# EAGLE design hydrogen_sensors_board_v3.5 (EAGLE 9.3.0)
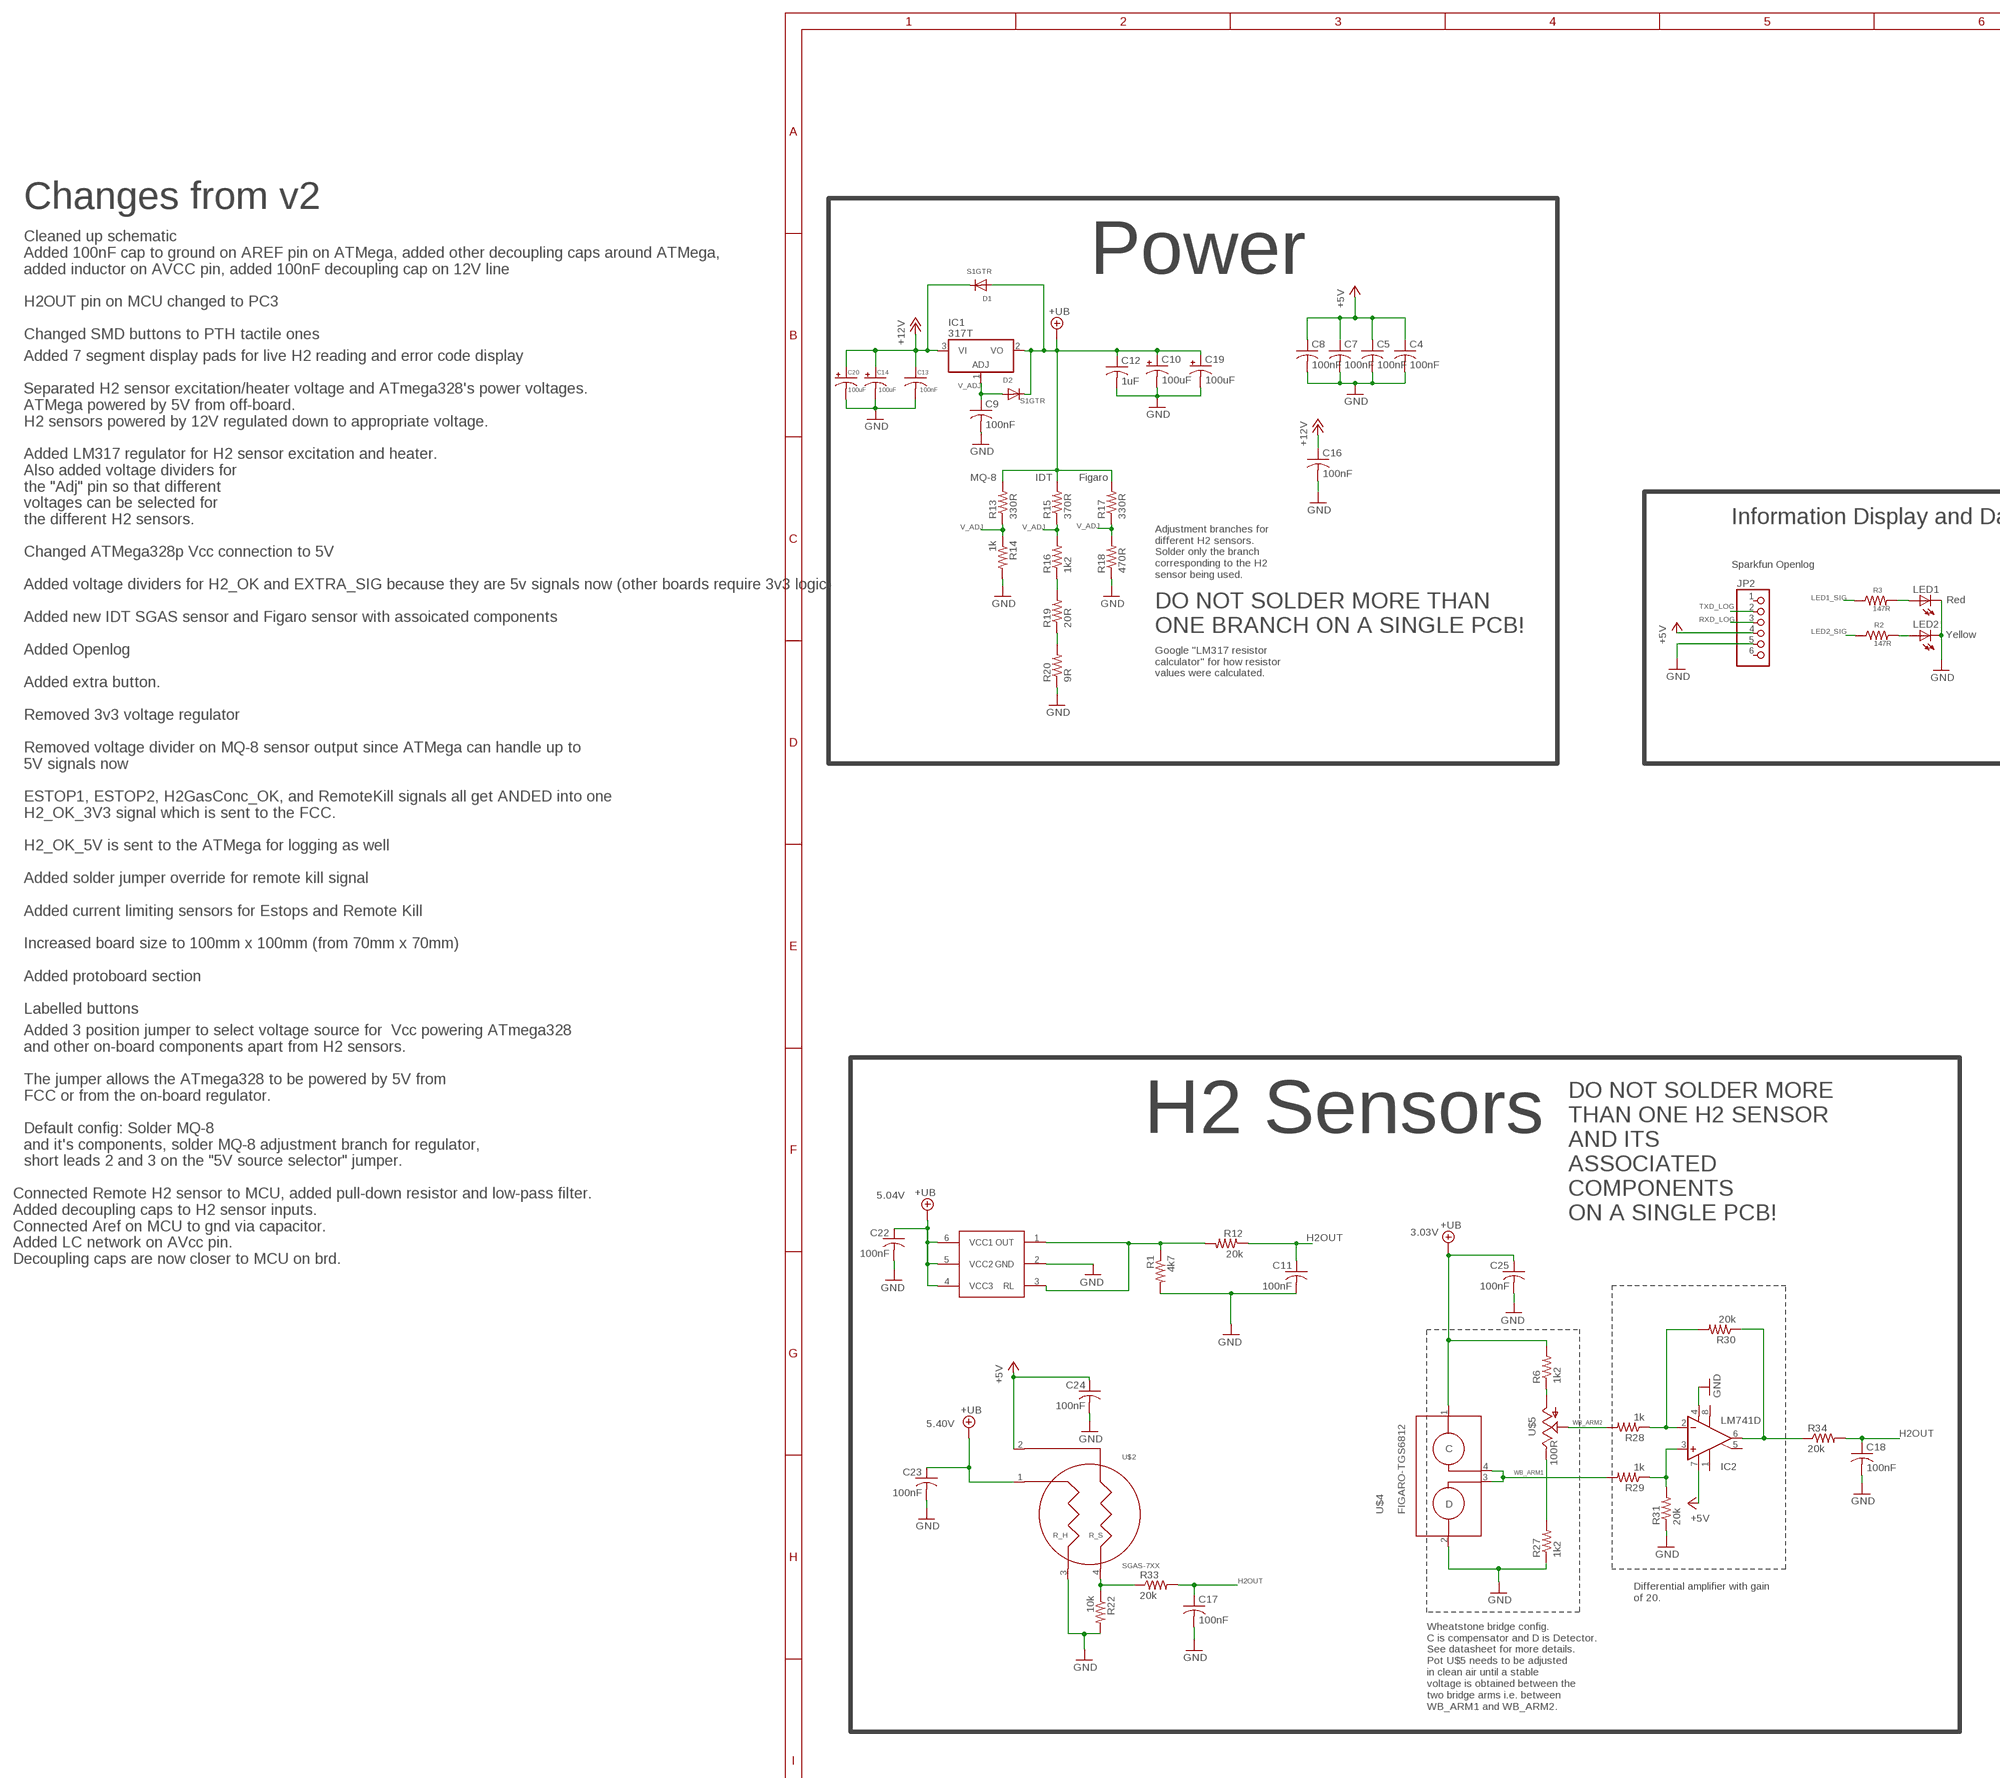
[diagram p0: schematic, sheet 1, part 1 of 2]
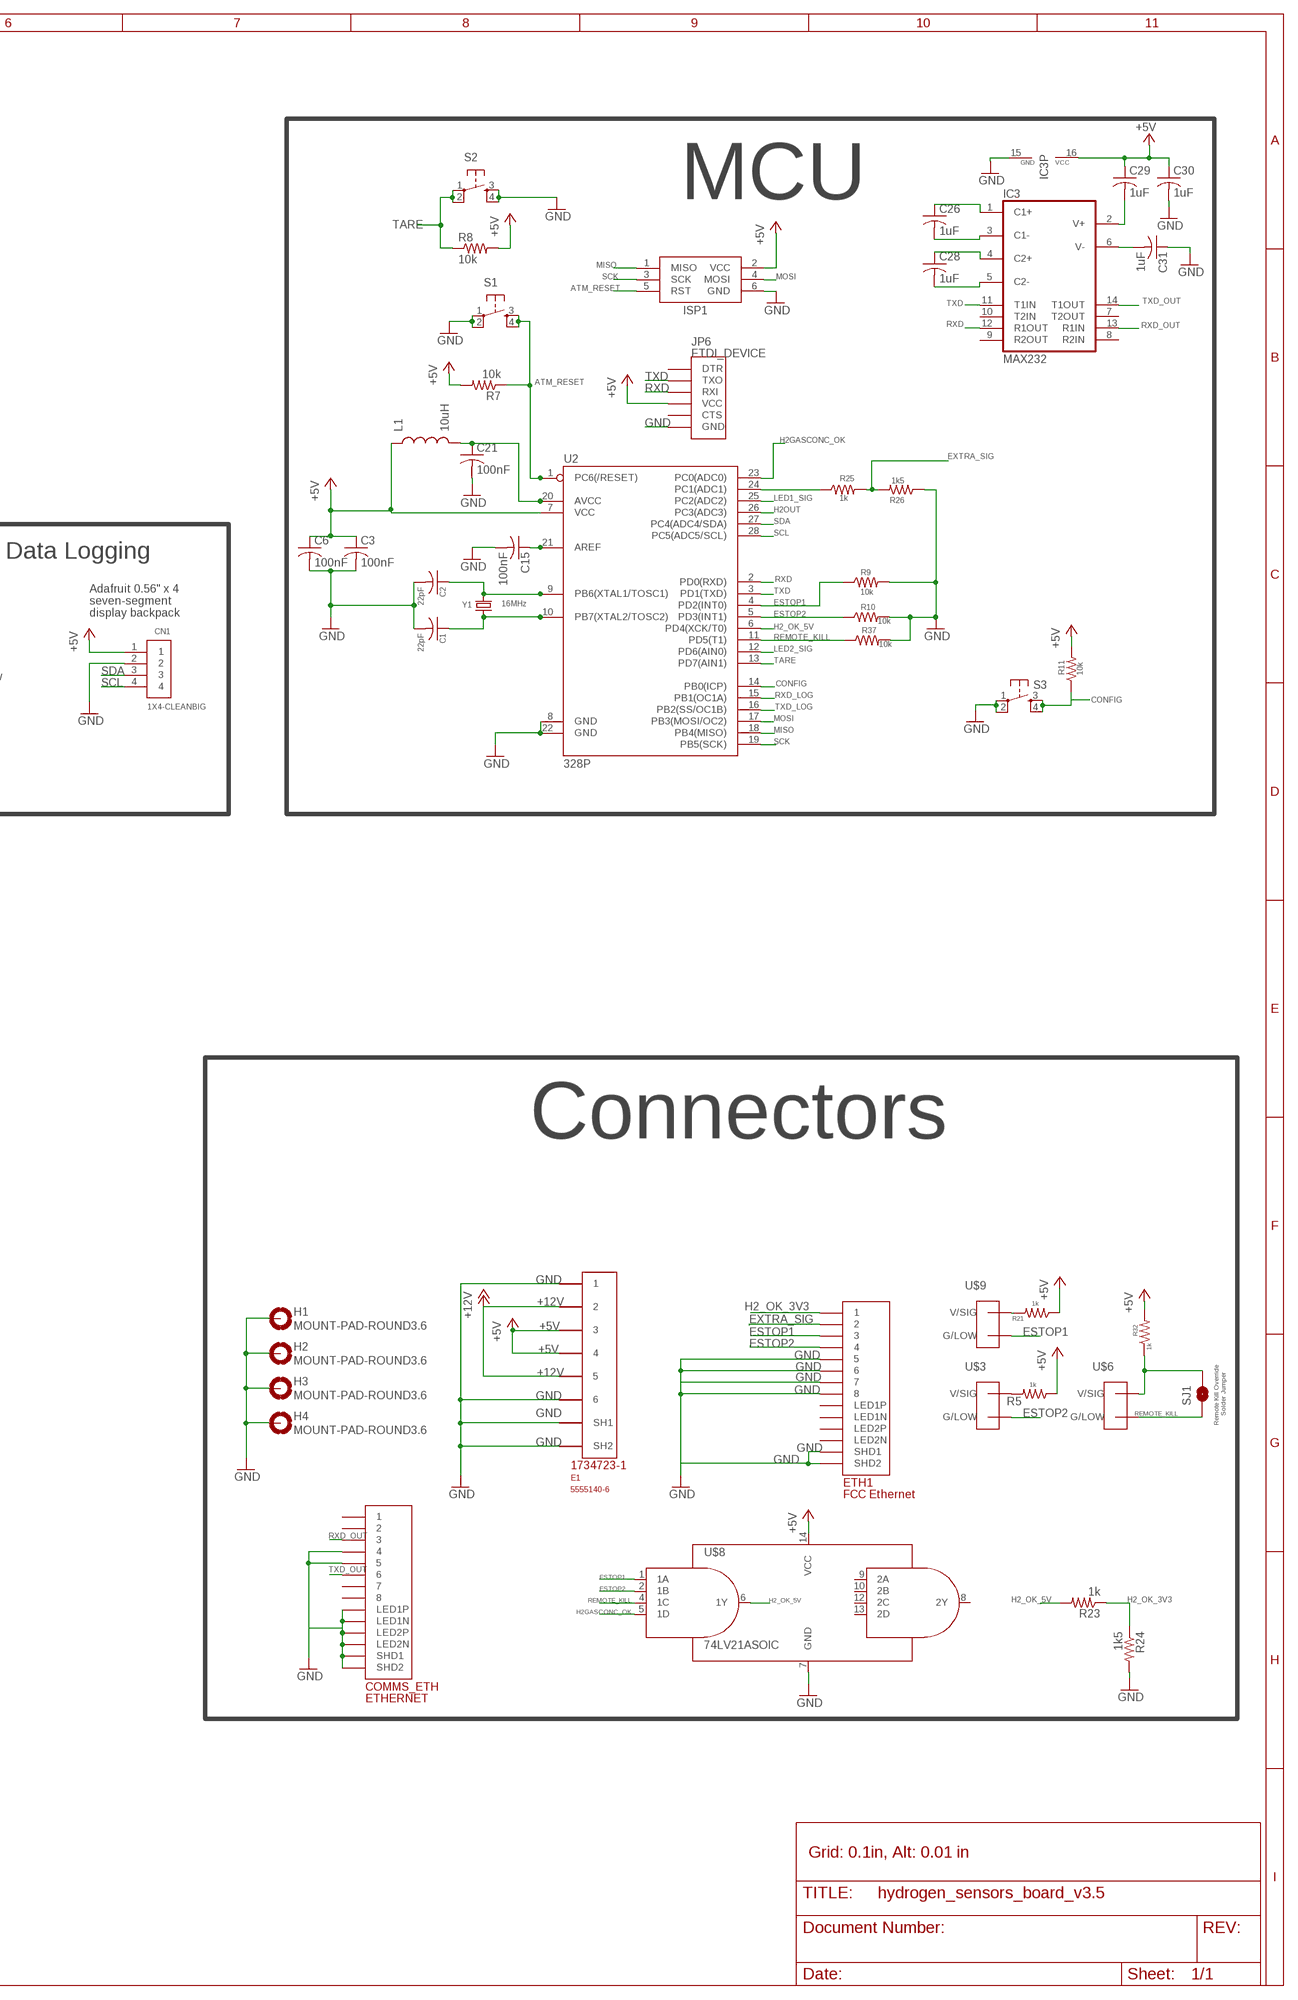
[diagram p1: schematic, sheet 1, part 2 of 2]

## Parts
C1  22pF  C-USC0603K  [C0603K]
C2  22pF  C-USC0603K  [C0603K]
C3  100nF  C-USC0603  [C0603]
C4  100nF  C-USC0603  [C0603]
C5  100nF  C-USC0603  [C0603]
C6  100nF  C-USC0603  [C0603]
C7  100nF  C-USC0603  [C0603]
C8  100nF  C-USC0603  [C0603]
C9  100nF  C-USC0603  [C0603]
C10  100uF  CPOL-USB/3528-21R  [B/3528-21R]
C11  100nF  C-USC0603  [C0603]
C12  1uF  C-USC0603  [C0603]
C13  100nF  C-USC0603  [C0603]
C14  100uF  CPOL-USB/3528-21R  [B/3528-21R]
C15  100nF  C-USC0603  [C0603]
C16  100nF  C-USC0603  [C0603]
C17  100nF  C-USC0603  [C0603]
C18  100nF  C-USC0603  [C0603]
C19  100uF  CAP_POLPTH1  [CPOL-RADIAL-100UF-25V]
C20  100uF  CAP_POLPTH1  [CPOL-RADIAL-100UF-25V]
C21  100nF  C-USC0603  [C0603]
C22  100nF  C-USC0603  [C0603]
C23  100nF  C-USC0603  [C0603]
C24  100nF  C-USC0603  [C0603]
C25  100nF  C-USC0603  [C0603]
C26  1uF  C-USC0603  [C0603]
C28  1uF  C-USC0603  [C0603]
C29  1uF  C-USC0603  [C0603]
C30  1uF  C-USC0603  [C0603]
C31  1uF  C-USC0603  [C0603]
CN1  1X4-CLEANBIG  [1X04-CLEANBIG]
COMMS_ETH  ETHERNET  [A122645-ND]
D1  S1GTR  DIODESMA  [SMADIODE]
D2  S1GTR  DIODESMA  [SMADIODE]
E1  5555140-6  [1734723-1_RJ11]
ETH1  FCC Ethernet  ETHERNET  [A122645-ND]
H1  MOUNT-PAD-ROUND3.6  [3,6-PAD]
H2  MOUNT-PAD-ROUND3.6  [3,6-PAD]
H3  MOUNT-PAD-ROUND3.6  [3,6-PAD]
H4  MOUNT-PAD-ROUND3.6  [3,6-PAD]
IC1  317T  [TO220H]
IC2  LM741D  [SO08]
IC3  MAX232  [DIL16]
ISP1  AVRISP-BOX  [AVRISP-BOX]
JP2  PINHD-1X6LOCK  [1X06-BIGLOCK]
JP6  FTDI_DEVICE  [FTDI_DEVICE_SIDE]
L1  10uH  INDUCTOR0603  [0603]
LED1  Red  LEDCHIPLED_0805  [CHIPLED_0805]
LED2  Yellow  LEDCHIPLED_0805  [CHIPLED_0805]
R1  4k7  RESISTOR0603-RES  [0603-RES]
R2  147R  RESISTOR0603-RES  [0603-RES]
R3  147R  RESISTOR0603-RES  [0603-RES]
R5  1k  RESISTOR0603-RES  [0603-RES]
R6  1k2  RESISTOR0603-RES  [0603-RES]
R7  10k  RESISTOR0603-RES  [0603-RES]
R8  10k  RESISTOR0603-RES  [0603-RES]
R9  10k  RESISTOR0603-RES  [0603-RES]
R10  10k  RESISTOR0603-RES  [0603-RES]
R11  10k  RESISTOR0603-RES  [0603-RES]
R12  20k  RESISTOR0603-RES  [0603-RES]
R13  330R  RESISTOR0603-RES  [0603-RES]
R14  1k  RESISTOR0603-RES  [0603-RES]
R15  370R  RESISTOR0603-RES  [0603-RES]
R16  1k2  RESISTOR0603-RES  [0603-RES]
R17  330R  RESISTOR0603-RES  [0603-RES]
R18  470R  RESISTOR0603-RES  [0603-RES]
R19  20R  RESISTOR0603-RES  [0603-RES]
R20  9R  RESISTOR0603-RES  [0603-RES]
R21  1k  RESISTOR0603-RES  [0603-RES]
R22  10k  RESISTOR0603-RES  [0603-RES]
R23  1k  RESISTOR0603-RES  [0603-RES]
R24  1k5  RESISTOR0603-RES  [0603-RES]
R25  1k  RESISTOR0603-RES  [0603-RES]
R26  1k5  RESISTOR0603-RES  [0603-RES]
R27  1k2  RESISTOR0603-RES  [0603-RES]
R28  1k  RESISTOR0603-RES  [0603-RES]
R29  1k  RESISTOR0603-RES  [0603-RES]
R30  20k  RESISTOR0603-RES  [0603-RES]
R31  20k  RESISTOR0603-RES  [0603-RES]
R32  1k  RESISTOR0603-RES  [0603-RES]
R33  20k  RESISTOR0603-RES  [0603-RES]
R34  20k  RESISTOR0603-RES  [0603-RES]
R37  10k  RESISTOR0603-RES  [0603-RES]
S1  TAC_SWITCHPTH  [TACTILE-PTH]
S2  TAC_SWITCHPTH  [TACTILE-PTH]
S3  TAC_SWITCHPTH  [TACTILE-PTH]
SJ1  SOLDERJUMPERNO  [SJ_2S-NO]
U2  328P  ATMEGA328P_PDIP  [DIP28]
U$1  MQ-8MQ-8  [MQ-8]
U$2  SGAS-7XX  [TO39]
U$3  TE770966  [2X1-MATE-N-LOCK]
U$4  FIGARO-TGS6812  [4PTH]
U$5  100R  POT100K_3362U  [3362U]
U$6  TE770966  [2X1-MATE-N-LOCK]
U$8  74LV21ASOIC  [SOIC-14]
U$9  TE770966  [2X1-MATE-N-LOCK]
Y1  16MHz  CRYSTALHC49US  [HC49US]

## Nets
+5V: C3.1 C4.1 C5.1 C6.1 C7.1 C8.1 C24.1 C29.1 C30.1 CN1.1 E1.3 E1.4 IC2.7(V+) IC3.16(VCC) ISP1.2(VCC) JP2.4 JP6.P$4(VCC) L1.1 R5.1 R7.2 R8.2 R11.2 R21.1 R32.2 U2.7(VCC) U$2.2 U$8.14(VCC)
+12V: C13.1 C14.+ C16.1 C20.1(+) D1.C E1.2 E1.5 IC1.3(VI)
+UB: C10.+ C12.1 C19.1(+) C22.1 C23.1 C25.1 D1.A D2.C IC1.2(VO) R6.2 R13.2 R15.2 R17.2 U$1.4(VCC3) U$1.5(VCC2) U$1.6(VCC1) U$2.1 U$4.1
ATM_RESET: ISP1.5(RST) R7.1 S1.3 S1.4 U2.1(PC6(/RESET))
CONFIG: R11.1 S3.3 S3.4 U2.14(PB0(ICP))
ESTOP1: ETH1.P$3 R9.1 U2.4(PD2(INT0)) U$8.1(1A) U$9.CIRCUIT2(G/LOW)
ESTOP2: ETH1.P$4 R10.1 U2.5(PD3(INT1)) U$3.CIRCUIT2(G/LOW) U$8.2(1B)
EXTRA_SIG: ETH1.P$2 R25.2 R26.2
GND: C1.2 C2.2 C3.2 C4.2 C5.2 C6.2 C7.2 C8.2 C9.2 C10.- C11.2 C12.2 C13.2 C14.- C15.2 C16.2 C17.2 C18.2 C19.2(-) C20.2(-) C21.2 C22.2 C23.2 C24.2 C25.2 C30.2 C31.1 CN1.2 COMMS_ETH.P$4 COMMS_ETH.P$5 COMMS_ETH.P$9(LED1N) COMMS_ETH.P$10(LED1P) COMMS_ETH.P$11(LED2N) COMMS_ETH.P$12(LED2P) COMMS_ETH.P$13(SHD1) COMMS_ETH.P$14(SHD2) E1.1 E1.6 E1.SH1 E1.SH2 ETH1.P$5 ETH1.P$6 ETH1.P$7 ETH1.P$8 ETH1.P$13(SHD1) ETH1.P$14(SHD2) H1.B3,6(MOUNT) H2.B3,6(MOUNT) H3.B3,6(MOUNT) H4.B3,6(MOUNT) IC2.4(V-) IC3.15(GND) ISP1.6(GND) JP2.5 JP6.P$6(GND) LED1.C LED2.C R1.2 R9.2 R10.2 R14.2 R18.1 R20.1 R22.2 R24.2 R26.1 R27.1 R31.1 R37.2 S1.1 S1.2 S2.3 S2.4 S3.1 S3.2 U2.8(GND) U2.22(GND) U$1.2(GND) U$2.3 U$4.2 U$8.7(GND)
H2_OK_3V3: ETH1.P$1 R23.1 R24.1
H2_OK_5V: R23.2 U2.6(PD4(XCK/T0)) U$8.6(1Y)
H2GASCONC_OK: U2.23(PC0(ADC0)) U$8.5(1D)
H2OUT: C11.1 C17.1 C18.1 R12.1 R33.2 R34.2 U2.26(PC3(ADC3))
LED1_SIG: R3.1 U2.25(PC2(ADC2))
LED2_SIG: R2.1 U2.12(PD6(AIN0))
MISO: ISP1.1(MISO) U2.18(PB4(MISO))
MOSI: ISP1.4(MOSI) U2.17(PB3(MOSI/OC2))
N$1: C2.1 U2.9(PB6(XTAL1/TOSC1)) Y1.2
N$2: R6.1 U$5.P$3(A)
N$3: C1.1 U2.10(PB7(XTAL2/TOSC2)) Y1.1
N$4: C15.1 U2.21(AREF)
N$5: R22.1 R33.1 U$2.4
N$6: LED2.A R2.2
N$7: LED1.A R3.2
N$10: R27.2 U$5.P$1(E)
N$11: R21.2 U$9.CIRCUIT1(V/SIG)
N$12: R25.1 U2.24(PC1(ADC1))
N$13: IC2.2(-IN) R28.1 R30.2
N$14: R16.1 R19.2
N$15: C29.2 IC3.2(V+)
N$16: C31.2 IC3.6(V-)
N$17: R19.1 R20.2
N$18: R1.1 R12.2 U$1.1(OUT) U$1.3(RL)
N$20: IC2.6(OUT) R30.1 R34.1
N$21: R5.2 U$3.CIRCUIT1(V/SIG)
N$22: IC2.3(+IN) R29.1 R31.2
N$24: R32.1 SJ1.2 U$6.CIRCUIT1(V/SIG)
N$62: C21.1 L1.2 U2.20(AVCC)
N$63: C26.1 IC3.1(C1+)
N$65: C26.2 IC3.3(C1-)
N$66: C28.1 IC3.4(C2+)
N$67: C28.2 IC3.5(C2-)
REMOTE_KILL: R37.1 SJ1.1 U2.11(PD5(T1)) U$6.CIRCUIT2(G/LOW) U$8.4(1C)
RXD: IC3.12(R1OUT) JP6.P$3(RXI) U2.2(PD0(RXD))
RXD_LOG: JP2.3 U2.15(PB1(OC1A))
RXD_OUT: COMMS_ETH.P$3 IC3.13(R1IN)
SCK: ISP1.3(SCK) U2.19(PB5(SCK))
SCL: CN1.4 U2.28(PC5(ADC5/SCL))
SDA: CN1.3 U2.27(PC4(ADC4/SDA))
TARE: R8.1 S2.1 S2.2 U2.13(PD7(AIN1))
TXD: IC3.11(T1IN) JP6.P$2(TXO) U2.3(PD1(TXD))
TXD_LOG: JP2.2 U2.16(PB2(SS/OC1B))
TXD_OUT: COMMS_ETH.P$6 IC3.14(T1OUT)
V_ADJ: C9.1 D2.A IC1.1(ADJ) R13.1 R14.1 R15.1 R16.2 R17.1 R18.2
WB_ARM1: R29.2 U$4.3 U$4.4
WB_ARM2: R28.2 U$5.P$2(S)
Unconnected: COMMS_ETH.P$1 COMMS_ETH.P$2 COMMS_ETH.P$7 COMMS_ETH.P$8 ETH1.P$9(LED1N) ETH1.P$10(LED1P) ETH1.P$11(LED2N) ETH1.P$12(LED2P) IC2.1(ON1) IC2.5(ON2) IC2.8(OPT) IC3.7(T2OUT) IC3.8(R2IN) IC3.9(R2OUT) IC3.10(T2IN) JP2.1 JP2.6 JP6.P$1(DTR) JP6.P$5(CTS) U$8.8(2Y) U$8.9(2A) U$8.10(2B) U$8.12(2C) U$8.13(2D)

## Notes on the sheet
- MCU
- Changes from v2
- Cleaned up schematic
  Added 100nF cap to ground on AREF pin on ATMega, added other decoupling caps around ATMega, 
  added inductor on AVCC pin, added 100nF decoupling cap on 12V line
- Power
- H2OUT pin on MCU changed to PC3
- Changed SMD buttons to PTH tactile ones
- Added 7 segment display pads for live H2 reading and error code display
- Separated H2 sensor excitation/heater voltage and ATmega328's power voltages.
  ATMega powered by 5V from off-board.
  H2 sensors powered by 12V regulated down to appropriate voltage.
- MQ-8 | IDT | Figaro
- Added LM317 regulator for H2 sensor excitation and heater.
  Also added voltage dividers for 
  the "Adj" pin so that different 
  voltages can be selected for
  the different H2 sensors.
- Information Display and Data Logging
- Changed ATMega328p Vcc connection to 5V
- Sparkfun Openlog
- Adafruit 0.56" x 4 
  seven-segment 
  display backpack
- Added voltage dividers for H2_OK and EXTRA_SIG because they are 5v signals now (other boards require 3v3 logic)
- Adjustment branches for 
  different H2 sensors. 
  Solder only the branch 
  corresponding to the H2 
  sensor being used.
- Added new IDT SGAS sensor and Figaro sensor with assoicated components
- DO NOT SOLDER MORE THAN
  ONE BRANCH ON A SINGLE PCB!
- Added Openlog
- Google "LM317 resistor 
  calculator" for how resistor 
  values were calculated.
- Added extra button.
- Removed 3v3 voltage regulator
- Removed voltage divider on MQ-8 sensor output since ATMega can handle up to 
  5V signals now
  
  ESTOP1, ESTOP2, H2GasConc_OK, and RemoteKill signals all get ANDED into one
  H2_OK_3V3 signal which is sent to the FCC.
- H2_OK_5V is sent to the ATMega for logging as well
- Added solder jumper override for remote kill signal
  
  Added current limiting sensors for Estops and Remote Kill
- Increased board size to 100mm x 100mm (from 70mm x 70mm)
  
  Added protoboard section
  
  Labelled buttons
- Connectors
- H2 Sensors
- Added 3 position jumper to select voltage source for  Vcc powering ATmega328
  and other on-board components apart from H2 sensors.
  
  The jumper allows the ATmega328 to be powered by 5V from 
  FCC or from the on-board regulator.
  
  Default config: Solder MQ-8 
  and it's components, solder MQ-8 adjustment branch for regulator, 
  short leads 2 and 3 on the "5V source selector" jumper.
- 5.04V
- DO NOT SOLDER MORE
  THAN ONE H2 SENSOR
  AND ITS 
  ASSOCIATED 
  COMPONENTS
  ON A SINGLE PCB!
- 3.03V
- Connected Remote H2 sensor to MCU, added pull-down resistor and low-pass filter.
  Added decoupling caps to H2 sensor inputs.
  Connected Aref on MCU to gnd via capacitor.
  Added LC network on AVcc pin.
  Decoupling caps are now closer to MCU on brd.
- Remote Kill Override 
  Solder Jumper
- 5.40V
- Differential amplifier with gain
  of 20.
- Wheatstone bridge config.
  C is compensator and D is Detector.
  See datasheet for more details.
  Pot U$5 needs to be adjusted
  in clean air until a stable
  voltage is obtained between the
  two bridge arms i.e. between
  WB_ARM1 and WB_ARM2.
- Grid: 0.1in, Alt: 0.01 in

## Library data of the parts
C1-C9 C11-C13 C15-C18 C21-C26 C28-C31 = adafruit:C-US: CAPACITOR, American symbol
C10 C14 = adafruit:CPOL-US: POLARIZED CAPACITOR, American symbol
C19 C20 = SparkFun-Capacitors:CAP_POL: Capacitor Polarized
CN1 = adafruit:1X4: 4-pin connector
COMMS_ETH ETH1 = ETHERNET:ETHERNET: Ethernet port with 2 leds. digikey number A122645-ND
D1 D2 = adafruit:DIODE: Diode
E1 = 5555140-6 RJ11:5555140-6
H1-H4 = holes:MOUNT-PAD-ROUND: MOUNTING PAD, round
IC1 = linear:*317: Positive VOLTAGE REGULATOR
IC2 = linear:*741: OP AMP
IC3 = maxim:MAX232: RS232 TRANSCEIVER; MF: MAXIM; MPN: MAX232ACPE+; OC_FARNELL: 9723773; OC_NEWARK: 68K4544; SPICEPREFIX: X
ISP1 = adafruit:AVRISP: AVR ISP HEADER Standard 6 pin header for AVR programming
JP2 = adafruit:PINHD-1X6: PIN HEADER
JP6 = SparkFun-Connectors:FTDI_DEVICE: Connector which mates to FTDI basic or FTDI cable.
L1 = SparkFun:INDUCTOR: Inductors
LED1 LED2 = adafruit:LED: LED
R1 R5 R6 R9-R12 R21-R24 R27-R34 R37 = SparkFun-Passives:RESISTOR: Resistor
R2 R3 R7 R8 R13-R20 R25 R26 = SparkFun-Resistors:RESISTOR: Resistor
S1-S3 = SparkFun:TAC_SWITCH: Momentary Switch Button commonly used for reset or general input. Spark Fun Electronics SKU : COM-00097
SJ1 = SparkFun:SOLDERJUMPER: Solder Jumper
U2 = SparkFun-IC-Microcontroller:ATMEGA328P_PDIP: Atmel 328P Through hole ATMEGA328P uC used in the Arduino 32kb flash, 1k EEPROM, 2k SRAM Datasheet SparkFun Products Storefront component: AVR 28 Pin 20MHz 32K 6A/D - ATMega328P (COM-09061) SparkFun Simon Says - Through-Hole Soldering Kit (KIT-10547) SparkFun Learn to Solder - Simon Says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; PROD_ID: IC-09136
U$1 = donny_library:MQ-8
U$2 = gas-sensors-adnan:SGAS-7XX: Device for IDT SGAS 7xx family of sensors (701/707/711). This device created for H2 sensor (701) but can be used for other sensors in this family as well. Package is T039 with 4 leads.
U$3 U$6 U$9 = Shell2013:TE770966
U$4 = gas-sensors-adnan:FIGARO-TGS6812: Device for Figaro TGS6812 sensor Connect in wheatstone bridge configuration - see datasheet. Element D is sensitive to combustble gases. Element C is a reference element and is not sensitive to combustible gases. Use a potentiometer to adjust resistance of parallel arm until it matches the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
U$5 = SparkFun:POT
U$8 = SparkFun-DigitalIC:74LV21A: Quad input two circuit AND gate SOIC-14 package SN74LV21
Y1 = SparkFun-FreqCtrl:CRYSTAL: Various standard crystals. Proven footprints.

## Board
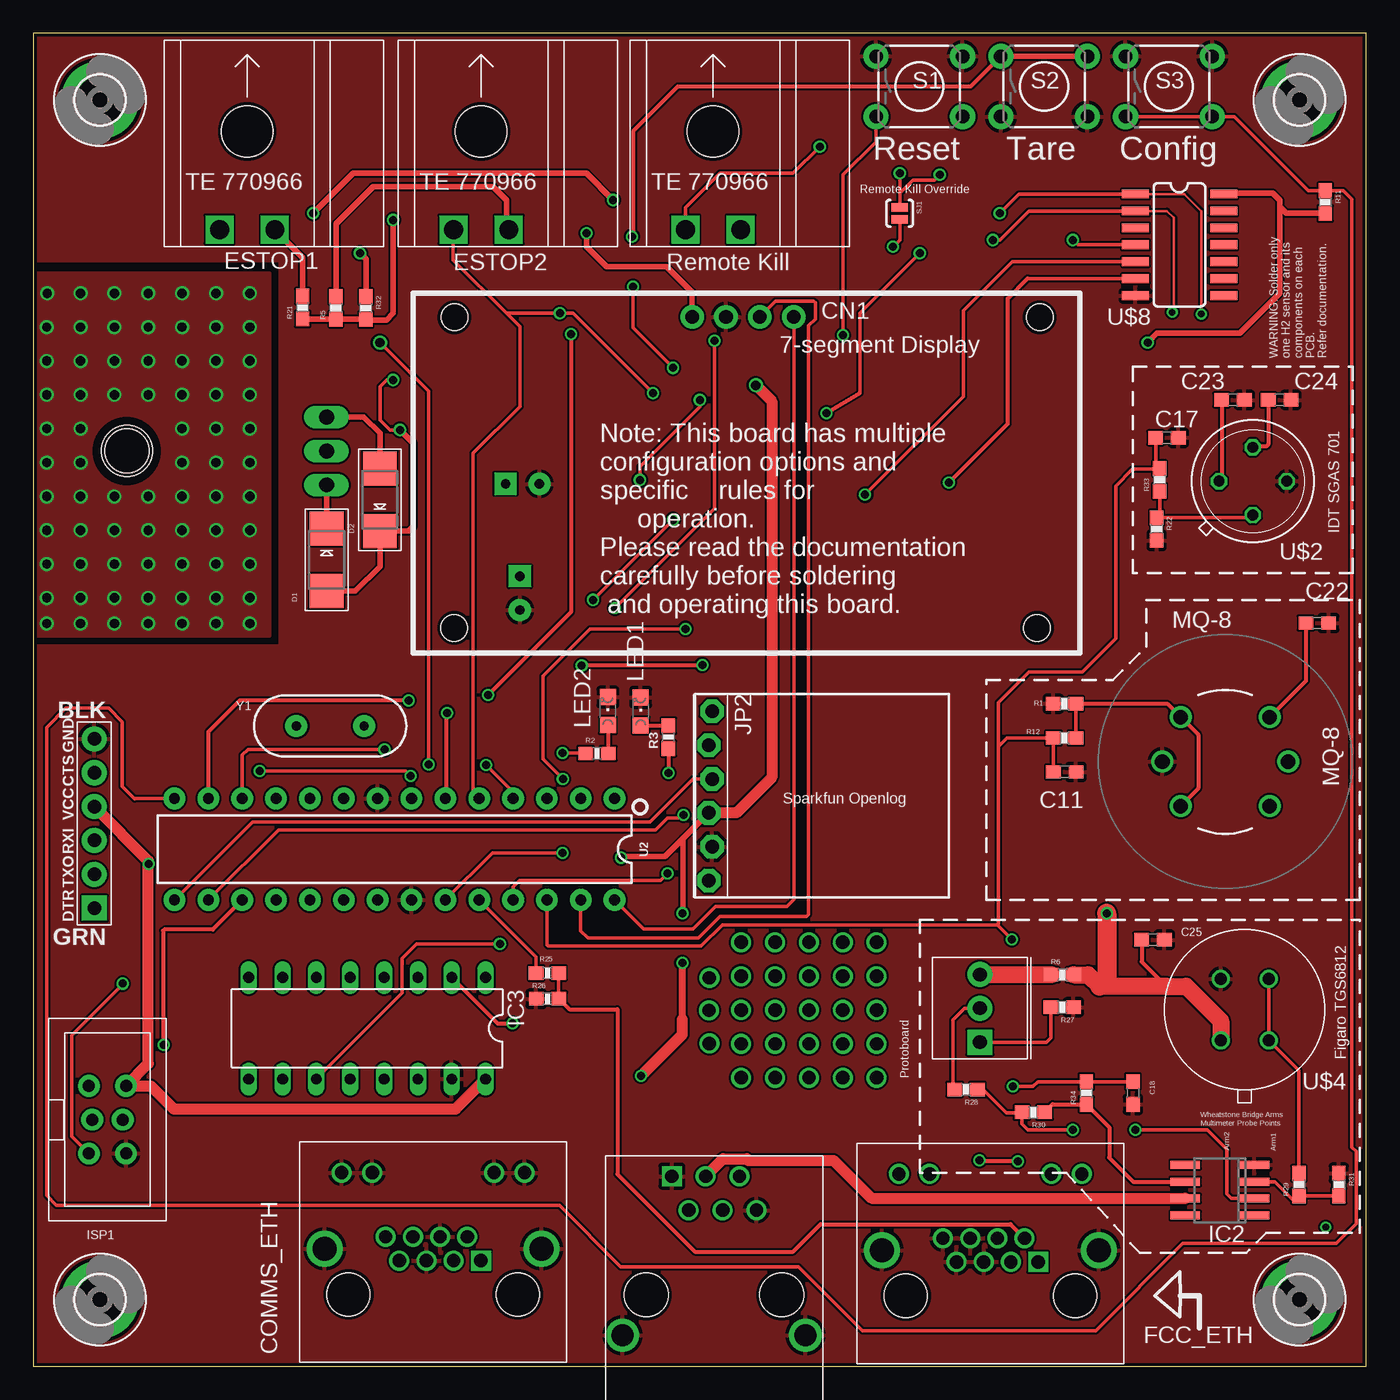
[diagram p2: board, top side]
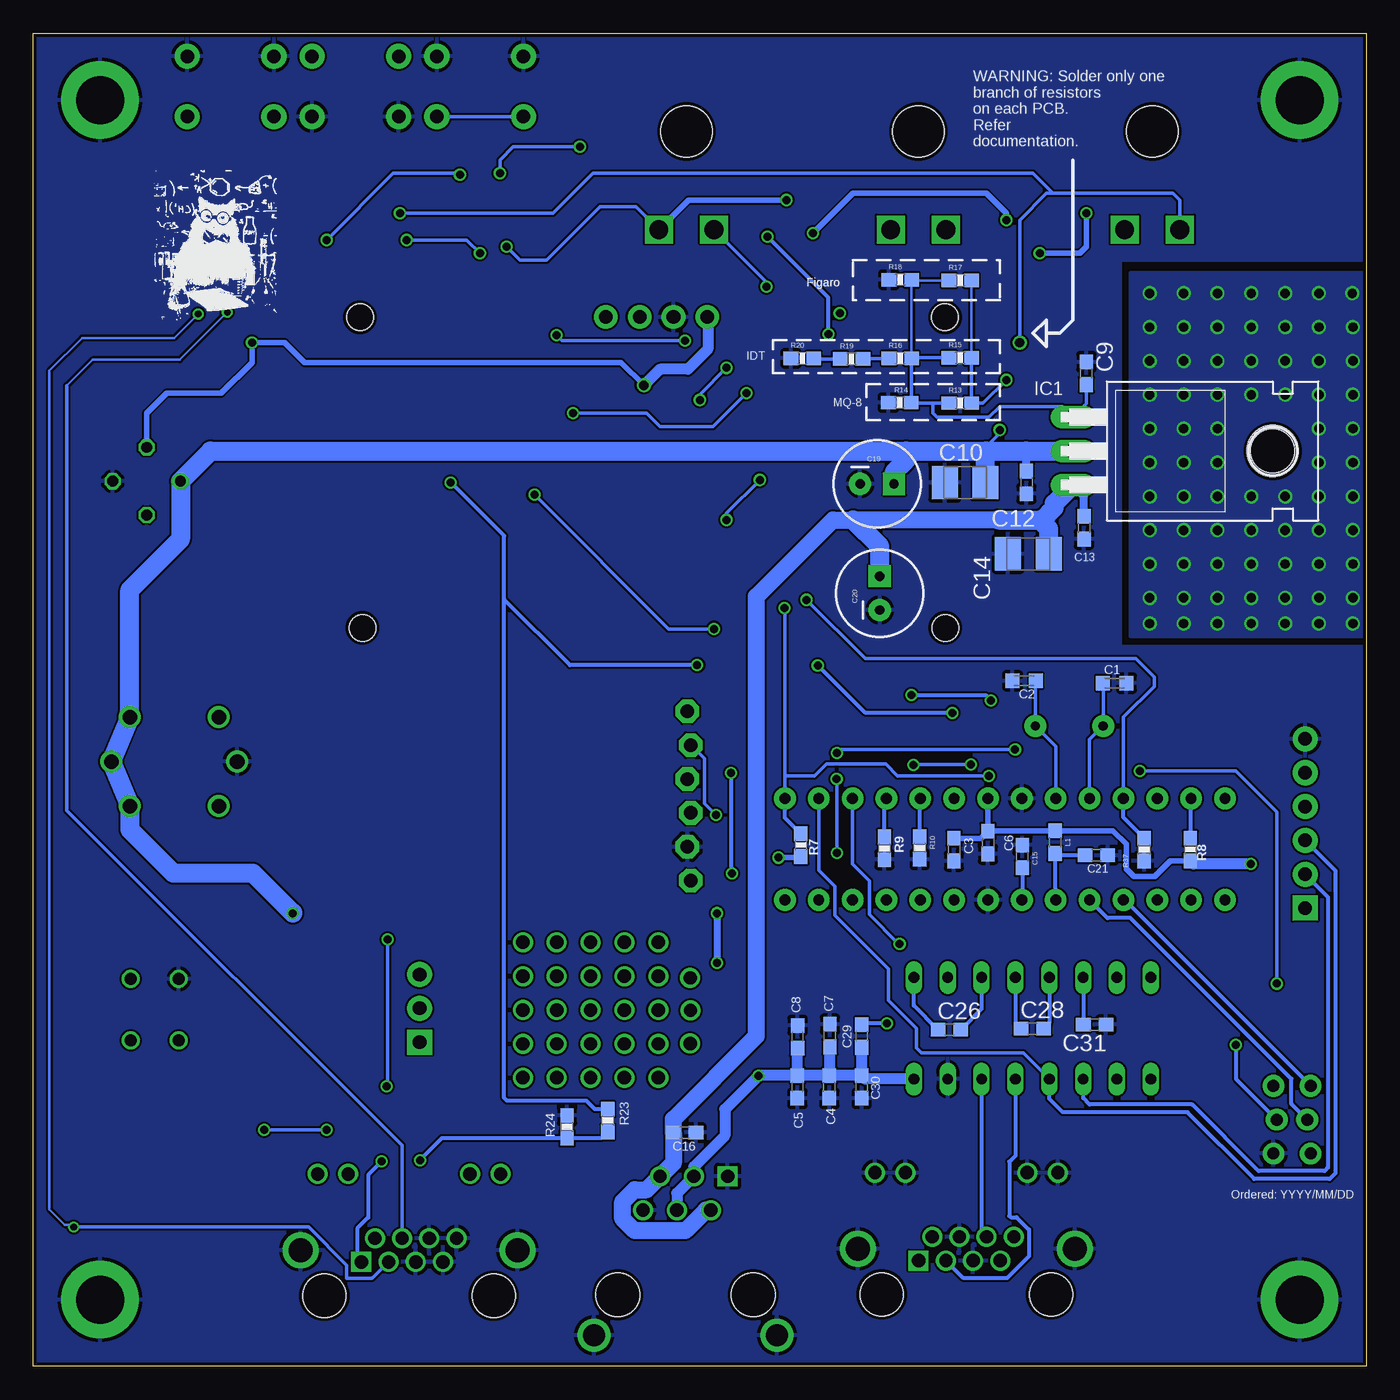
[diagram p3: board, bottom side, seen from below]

Size 100 x 100 mm. Coordinates in mm from the lower left corner, seen from the top.
Outline: 0,0 100,0 100,100 0,100 0,0
Copper layers (1*16): Top 0.035mm / dielectric 1.5mm / Bottom 0.035mm
Design rules "JLCPCB2Layer": minimum track width 6mil, minimum drill 10mil, track to track 6mil, track to pad 6mil, pad to pad 6mil, via to via 6mil, smd to smd 0mil, copper to edge 10mil, drill to drill 10mil, minimum pad ring 6mil, minimum via ring 6mil, stop-mask expansion 2mil, vias tented up to drill 100mil, thermal gap 10mil
Holes 2 mm at 31.6,78.7 75.5,78.7 75.3,55.39 31.58,55.39
Holes 3.84 mm at 7.01,68.67

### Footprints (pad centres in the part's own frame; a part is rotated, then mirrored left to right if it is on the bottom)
C0603K = smd 1.05 x 1.08: 1 -0.875,0; 2 0.875,0
C0603 = smd 1.1 x 1: 1 -0.85,0; 2 0.85,0
B/3528-21R = smd 1.95 x 2.5: + 1.525,0; - -1.525,0
CPOL-RADIAL-100UF-25V = drill 0.7 pad 1.651 square: 1 1.27,0 | drill 0.7 pad 1.651: 2 -1.27,0
1X04-CLEANBIG = drill 1.016 pad 1.778: 1 -3.81,0; 2 -1.27,0; 3 1.27,0; 4 3.81,0
A122645-ND = drill 1 square: P$1 3.58,2.54 | drill 1: P$2 2.56,4.32; P$3 1.54,2.54; P$4 0.52,4.32; P$5 -0.5,2.54; P$6 -1.52,4.32; P$7 -2.54,2.54; P$8 -3.56,4.32; P$9 -6.86,9.14; P$10 -4.57,9.14; P$11 4.57,9.14; P$12 6.86,9.14 | drill 1.8: P$13 -8.13,3.43; P$14 8.13,3.43 | hole 3.25: -6.35,0; 6.35,0
SMADIODE = smd 2.54 x 2.54: A 2.349,0; C -2.349,0
1734723-1_RJ11 = drill 1 square: 1 -3.81,2.54 | drill 1: 2 -2.54,0; 3 -1.27,2.54; 4 0,0; 5 1.27,2.54; 6 2.54,0 | drill 1.65: SH1 -7.5,-9.4; SH2 6.22,-9.4 | hole 3.3: -5.72,-6.35; 4.44,-6.35
3,6-PAD = drill 3.6 pad 5.842: B3,6 0,0
TO220H = drill 1.118 long: 1 -2.54,-10.16; 2 0,-10.16; 3 2.54,-10.16 | hole 3.302: 0,4.826
SO08 = smd 0.6 x 2.2: 1 -1.905,-2.6; 2 -0.635,-2.6; 3 0.635,-2.6; 4 1.905,-2.6; 5 1.905,2.6; 6 0.635,2.6; 7 -0.635,2.6; 8 -1.905,2.6
DIL16 = drill 0.813 long: 1 -8.89,-3.81; 2 -6.35,-3.81; 3 -3.81,-3.81; 4 -1.27,-3.81; 5 1.27,-3.81; 6 3.81,-3.81; 7 6.35,-3.81; 8 8.89,-3.81; 9 8.89,3.81; 10 6.35,3.81; 11 3.81,3.81; 12 1.27,3.81; 13 -1.27,3.81; 14 -3.81,3.81; 15 -6.35,3.81; 16 -8.89,3.81
AVRISP-BOX = drill 0.9 pad 1.626: 1 -1.397,2.54; 2 1.397,2.54; 3 -1.143,0; 4 1.143,0; 5 -1.397,-2.54; 6 1.397,-2.54
1X06-BIGLOCK = drill 1.016 pad 1.778 octagon: 1 -6.35,0.127; 2 -3.81,-0.127; 3 -1.27,0.127; 4 1.27,-0.127; 5 3.81,0.127; 6 6.35,-0.127
FTDI_DEVICE_SIDE = drill 1.016 pad 1.88 square: P$1 -6.35,0 | drill 1.016 pad 1.88: P$2 -3.81,0; P$3 -1.27,0; P$4 1.27,0; P$5 3.81,0; P$6 6.35,0
0603 = smd 1.1 x 1: 1 -0.85,0; 2 0.85,0
CHIPLED_0805 = smd 1.2 x 1.2: A 0,-1.05; C 0,1.05
0603-RES = smd 1.1 x 1: 1 -0.85,0; 2 0.85,0
TACTILE-PTH = drill 1.016 pad 1.88: 1 -3.251,2.261; 2 3.251,2.261; 3 -3.251,-2.261; 4 3.251,-2.261
SJ_2S-NO = smd 0.635 x 1.27: 1 -0.45,0; 2 0.45,0
DIP28 = drill 0.813 pad 1.626: 1 -16.51,-3.81; 2 -13.97,-3.81; 3 -11.43,-3.81; 4 -8.89,-3.81; 5 -6.35,-3.81; 6 -3.81,-3.81; 7 -1.27,-3.81; 8 1.27,-3.81; 9 3.81,-3.81; 10 6.35,-3.81; 11 8.89,-3.81; 12 11.43,-3.81; 13 13.97,-3.81; 14 16.51,-3.81; 15 16.51,3.81; 16 13.97,3.81; 17 11.43,3.81; 18 8.89,3.81; 19 6.35,3.81; 20 3.81,3.81; 21 1.27,3.81; 22 -1.27,3.81; 23 -3.81,3.81; 24 -6.35,3.81; 25 -8.89,3.81; 26 -11.43,3.81; 27 -13.97,3.81; 28 -16.51,3.81
MQ-8 = drill 1.1: 1 -3.337,3.337; 2 -4.72,0; 3 -3.337,-3.337; 4 3.337,-3.337; 5 4.72,0; 6 3.337,3.337
TO39 = drill 0.813 octagon: 1 -2.54,0; 2 0,2.54; 3 2.54,0; 4 0,-2.54
2X1-MATE-N-LOCK = drill 1.4 square: CIRCUIT1 -2.07,14.23; CIRCUIT2 2.07,14.23 | hole 3.86: 0,6.86
4PTH = drill 0.9: 1 -1.8,-2.3; 2 -1.8,2.3; 3 1.8,2.3; 4 1.8,-2.3
3362U = drill 1.016 pad 1.88 square: P$1 0,2.54 | drill 1.016 pad 1.88: P$2 2.54,2.54; P$3 5.08,2.54
SOIC-14 = smd 0.66 x 2.032: 1 -4.445,-3.315; 2 -3.175,-3.315; 3 -1.905,-3.315; 4 -0.635,-3.315; 5 0.635,-3.315; 6 1.905,-3.315; 7 3.175,-3.315; 8 3.175,3.315; 9 1.905,3.315; 10 0.635,3.315; 11 -0.635,3.315; 12 -1.905,3.315; 13 -3.175,3.315; 14 -4.445,3.315
HC49US = drill 0.7 pad 1.651: 1 -2.54,0; 2 2.54,0

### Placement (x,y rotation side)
C1  18.86,51.25 0 bottom
C2  25.66,51.42 180 bottom
C3  30.93,38.76 270 bottom
C4  40.28,20.96 270 bottom
C5  42.68,20.95 270 bottom
C6  28.38,39.29 270 bottom
C7  40.23,24.81 90 bottom
C8  42.66,24.71 90 bottom
C9  21,74.5 90 bottom
C10  30.1,66.3 0 bottom
C11  77.38,44.59 0 top
C12  25.49,66.31 270 bottom
C13  21.17,62.91 270 bottom
C14  25.35,60.95 0 bottom
C15  25.8,38.24 90 bottom
C16  51.13,17.53 0 bottom
C17  85.05,69.65 0 top
C18  82.5,20.5 270 top
C19  36.7,66.2 0 bottom
C20  36.5,58 90 bottom
C21  20.24,38.33 0 bottom
C22  96.33,55.75 0 top
C23  90,72.5 0 top
C24  93.5,72.5 0 top
C25  84,32 0 top
C26  31.27,25.25 0 bottom
C28  25.04,25.32 0 bottom
C29  37.85,24.77 90 bottom
C30  37.85,20.95 270 bottom
C31  20.37,25.63 180 bottom
CN1  53.24,78.72 0 top
COMMS_ETH  30,5.38 0 top
D1  22,60.5 270 top
D2  26,65 90 top
E1  51.71,11.71 0 top
ETH1  71.81,5.28 0 top
H1  5,95 0 top
H2  95,95 0 top
H3  95,5 0 top
H4  5,5 0 top
IC1  11.84,68.66 270 bottom
IC2  89.02,13.21 90 top
IC3  25.04,25.35 180 top
ISP1  5.56,18.49 0 top
JP2  50.8,42.78 270 top
JP6  4.57,40.72 90 top
L1  23.35,39.31 270 bottom
LED1  45.57,49.12 0 top
LED2  43.1,49.15 0 top
R1  77.37,49.7 180 top
R2  42.29,45.97 0 top
R3  47.65,47.2 90 top
R5  22.7,79.4 90 top
R6  77.21,29.37 0 top
R7  42.41,39.1 270 bottom
R8  13.19,38.76 270 bottom
R9  36.15,38.86 270 bottom
R10  33.49,38.88 270 bottom
R11  96.94,87.34 270 top
R12  77.37,47.13 0 top
R13  30.46,72.25 0 bottom
R14  35,72.3 180 bottom
R15  30.46,75.66 0 bottom
R16  34.96,75.61 0 bottom
R17  30.46,81.46 0 bottom
R18  34.96,81.51 0 bottom
R19  38.61,75.56 0 bottom
R20  42.31,75.62 0 bottom
R21  20.21,79.43 90 top
R22  84.28,62.81 270 top
R23  56.9,18.43 90 bottom
R24  59.96,17.96 90 bottom
R25  38.57,29.5 0 top
R26  38.58,27.57 0 top
R27  77.19,26.93 180 top
R28  69.98,20.76 180 top
R29  94.96,13.62 90 top
R30  75.03,19.05 180 top
R31  97.95,13.63 270 top
R32  24.95,79.39 270 top
R33  84.5,66.5 90 top
R34  79,20.5 90 top
R37  16.66,38.76 270 bottom
S1  66.47,96.02 0 top
S2  75.84,96.02 0 top
S3  85.2,96.02 0 top
SJ1  65,86.5 270 top
U2  27.1,38.79 180 top
U$1  89.42,45.36 0 top
U$2  91.5,66.4 0 top
U$3  33.6,99.5 180 top
U$4  90.88,26.75 0 top
U$5  73.56,24.31 90 top
U$6  51,99.5 180 top
U$8  86,83.5 270 top
U$9  16.05,99.5 180 top
Y1  22.28,48.03 0 top

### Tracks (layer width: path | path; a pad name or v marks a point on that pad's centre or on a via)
+5V  (via drill 0.6, 0.7)
  Top 0.254: 89.37,88 U$8.14
  Top 0.305: C24.1 92.65,69.15 92.5,69 91.56,69 U$2.2
  Top 0.406: CN1.1 49.4,78.75 49.4,80.6 47.5,82.5 43,82.5 41.5,84 v41.5,85 | 93.5,87 93.5,80.5 90.5,77.5 84.3,77.5 v83.6,76.8 | 93.5,87 93.5,87.5 93,88 89.37,88 | 93.5,87 94.01,86.49 R11.2 | R21.1 20.24,78.55 R5.1 R32.2 24.99,78.5 26.5,78.5 27,79 v27,86 | JP2.4 48.74,39.58 | 48.74,39.58 47.39,38.23 44.09,38.23 v44.09,38.15 | 48.74,39.58 48.74,34.13 48.72,34.11 v48.72,33.98
  Top 0.508: 48.69,26.01 v48.69,30.25
  Top 0.813: v54.2,73.6 55.4,72.4 55.4,44.17 52.74,41.51 JP2.4 | 8.64,37.64 v8.66,37.67 | 8.64,37.64 8.64,22.71 ISP1.2 8.81,21.03 10.54,19.3 31.7,19.3 IC3.16 | E1.3 51.75,15.56 53.53,15.56 53.64,15.44 60.05,15.44 62.89,12.6 86.4,12.6 IC2.7 | JP6.P$4 8.64,37.92 8.64,37.64 | v45.59,21.79 48.69,24.89 48.69,26.01
  Bottom 0.406: 49.4,78.69 CN1.1 | v54.2,73.6 55.9,75.3 79.65,75.3 81.15,76.8 v83.6,76.8 83.6,75.3 85.9,73 90,73 91.5,71.5 U$2.2 | v27,86 27,86.5 28.5,88 38.5,88 v41.5,85 | C6.1 28.35,40.16 L1.1 19,40.16 18.01,39.17 18.01,37.31 17.45,36.75 15.85,36.75 14.7,37.91 R8.2 | C6.1 U2.7 | C6.1 28.91,39.6 C3.1 | v44.09,38.15 42.51,38.15 R7.2 | 48.72,30.28 v48.69,30.25
  Bottom 0.508: v48.72,33.98 48.72,30.28
  Bottom 0.813: 49.4,78.69 49.4,76.3 50.9,74.8 53,74.8 v54.2,73.6 | C30.1 C29.1 | C4.1 40.23,21.85 C7.1 | E1.4 51.71,12.98 E1.3 50.44,14.96 48.11,17.3 48.11,19.28 v45.59,21.79 v45.59,21.8 C5.1 | v8.66,37.67 12.95,37.67 R8.2 | IC3.16 37.58,21.54 C30.1 | C30.1 C4.1 | C4.1 C5.1 | C5.1 42.68,23.84 C8.1
+12V
  Top 0.406: D1.C IC1.3
  Bottom 0.61: C13.1 21.17,65.3 IC1.3
  Bottom 1.27: 27.6,63.5 38.5,63.5 40,63.5 45.74,57.76 45.74,24.77 51.98,18.53 C16.1 51.98,15.25 E1.5 53.99,13.25 54.89,13.25 55.79,12.35 55.79,11.07 54.89,10.17 51.08,10.17 49.54,11.71 E1.2
  Bottom 1.422: 27.6,63.5 24.5,63.5 | 24.5,63.5 24.3,63.5 23.4,64.4 23.4,64.72 IC1.3 | C14.+ 23.82,62.83 24.5,63.5 | C20.1 36.5,61.5 38.5,63.5
+UB  (via drill 0.6)
  Top 0.254: v27,74 26.5,74 26,73.5 26,71 26.75,70.25 v27.5,70.25
  Top 0.305: C23.1 89.15,66.59 U$2.1 | C22.1 95.48,51.42 U$1.6 | C25.1 83.15,30.35 85,28.5
  Top 0.406: v27.5,70.25 28.5,69.25 28.5,63 28.15,62.65 D2.C 26,60 24.15,58.15 D1.A
  Top 1.27: R6.2 79.13,29.37 80,28.5 85,28.5 86.5,28.5 89.08,25.92 U$4.1
  Top 1.422: v80.54,33.98 80.54,29.04 80,28.5
  Bottom 0.203: R17.2 R15.2
  Bottom 0.254: R15.2 R13.2 28.75,72.25 v27,74 | v27.5,70.25 27.5,70 28.5,69 28.5,68.66
  Bottom 0.61: C12.1 25.5,68.66
  Bottom 1.422: 34.5,68.66 86.7,68.66 U$2.1 88.96,62.04 92.76,58.24 U$1.6 U$1.5 U$1.4 92.76,40.26 89.5,37 83.53,37 80.54,34.01 v80.54,33.98 | 34.5,68.66 28.5,68.66 | 28.5,68.66 25.5,68.66 IC1.2 | C10.+ 28.57,68.58 28.5,68.66 | C19.1 35.43,67.07 34.5,68 34.5,68.66
ATM_RESET  (via drill 0.6)
  Top 0.254: S1.3 63.2,93.73 63.2,91.82 60.76,89.38 v60.76,77.37 | v43.64,56.87 51.1,64.34 v51.1,76.94 | ISP1.5 2.87,17.25 2.87,24.82 6.71,28.65 v6.71,28.7 | v16.97,44.65 27.94,44.65 v28.3,44.3
  Bottom 0.254: S1.4 S1.3 | U2.1 43.61,44.25 | 43.61,44.25 43.61,56.79 43.69,56.87 v43.64,56.87 | v51.1,76.94 60.33,76.94 v60.76,77.37 | v6.71,28.7 6.71,41.58 9.78,44.65 v16.97,44.65 | 43.61,44.25 43.56,44.3 41.38,44.3 40.49,45.19 36.04,45.19 35.15,44.3 v28.3,44.3
  Bottom 0.305: R7.1 43.61,41.15 U2.1
CONFIG
  Top 0.254: S3.3 S3.4 90.09,93.75 95.66,88.19 R11.1 98.3,88.19 98.93,87.55 98.93,16.43 99.24,16.13 99.24,10.69 97.77,9.22 86.26,9.22 79.7,2.67 62.2,2.67 57.4,7.47 44.07,7.47 39.47,12.06 1.73,12.06 0.99,12.8 0.99,47.93 2.44,49.38 5.64,49.38 6.68,48.34 6.68,43.48 7.62,42.55 7.67,42.6 U2.14
ESTOP1  (via drill 0.51, 0.6, 0.7)
  Top 0.203: U$8.1 86.35,87.94 87.63,86.67 v87.63,78.94
  Top 0.254: U$8.1 73.94,87.94 v72.5,86.5 | v26,76.8 29.65,73.15 29.65,45.15 v29.67,45.14 | v33.96,45.11 35.99,43.08 U2.4
  Bottom 0.203: v87.63,78.94 89.43,77.14 96.34,77.14 98.81,74.68 98.81,11.79 97.64,10.62 97.16,10.62 v96.98,10.44
  Bottom 0.254: v26,76.8 26,86 24,88 23.5,88 | 23.5,88 14.5,88 14,87.5 14,85.29 U$9.CIRCUIT2 | v72.5,86.5 61,86.5 58,89.5 25,89.5 23.5,88 | v96.98,10.44 79.35,10.44 76.48,7.57 76.48,6.58 74.59,6.58 ETH1.P$3 | v29.67,45.14 33.93,45.14 v33.96,45.11
  Bottom 0.305: R9.1 36.15,42.44 U2.4
ESTOP2  (via drill 0.51, 0.6)
  Top 0.203: U$8.2 85.05,86.67 85.57,86.16 85.57,79.2 v85.45,79.07
  Top 0.254: 35.5,79 36.5,78 36.5,72 33,68.5 33,43.05 U2.5 | 35.5,79 31.5,83 31.5,85.24 U$3.CIRCUIT2 | U$8.2 74.67,86.67 72.5,84.5 v72,84.5 | 35.5,79 v39.5,79 40.5,79 v46.5,73 | v66.5,83.5 62,79 62,73 v59.5,71.5
  Bottom 0.203: v85.45,79.07 89,75.51 95.53,75.51 97.48,73.56
  Bottom 0.254: v66.5,83.5 67.5,84.5 v72,84.5 | v46.5,73 49,70.5 53,70.5 54,71.5 v59.5,71.5 | 97.48,73.56 97.48,41.71 72.33,16.55 ETH1.P$4
  Bottom 0.305: R10.1 33.49,42.55 U2.5
EXTRA_SIG
  Top 0.254: R25.2 39.42,27.57 R26.2
  Top 0.305: R26.2 40.22,26.77 43.81,26.77 43.81,14.4 49.63,8.59 57,8.59 59.07,10.65 73.31,10.65 ETH1.P$2
GND
  pour Bottom: 0,100 0,83 18.5,83 18.5,54 0,54 0,0 100,0 100,100
  pour Top: 0,100 0,83 18.5,83 18.5,54 0,54 0,0 100,0 100,100
H2_OK_3V3  (via drill 0.6)
  Top 0.305: v70.97,15.44 71.02,15.39 73.86,15.39 v73.86,15.37
  Bottom 0.305: v70.97,15.44 70.97,15.49 69.36,17.11 R24.1 57.38,17.11 R23.1 | v73.86,15.37 74.88,14.35 74.88,11.15 75.69,10.34 75.69,8.12 ETH1.P$1
H2_OK_5V  (via drill 0.6)
  Top 0.254: U$8.6 74.6,81.59
  Top 0.305: 74.6,81.59 73.1,80.1 73.1,70.71 v68.68,66.29 | U2.6 31.01,42.7 31.01,49.05 v31.04,49.02 | v50.19,52.6 50.16,52.58 v41.15,52.58
  Bottom 0.305: R23.2 57.86,19.28 58.5,19.91 64.47,19.91 64.67,20.12 64.67,57.53 | 64.67,57.53 64.67,62.31 68.66,66.29 v68.68,66.29 | v31.04,49.02 37.57,49.02 41.12,52.58 v41.15,52.58 | v50.19,52.6 59.74,52.6 64.67,57.53
H2GASCONC_OK  (via drill 0.6)
  Top 0.254: U2.23 34.44,38.51 v39.7,38.51 | v39.73,44.04 38.23,45.54 38.23,51.77 41.78,55.32 v48.92,55.32 | v62.41,65.38 69.77,72.75 69.77,79.2 73.44,82.86 U$8.5
  Bottom 0.254: v39.7,38.51 39.7,44.02 v39.73,44.04 | v48.92,55.32 52.35,55.32 v62.41,65.38
H2OUT  (via drill 0.6)
  Top 0.254: 72.4,46.5 73.03,47.12 R12.1 C11.1 | 72.4,46.5 72.4,49.8 74.7,52.1 78.7,52.1 81.2,54.6 81.2,66.05 82.45,67.3 84.45,67.3 R33.2 84.2,67.65 C17.1 | v73.5,21 75,21 75.35,21.35 R34.2 C18.1 | U2.26 38.53,31.62 38.63,31.52 50.09,31.52 51.69,33.12 72.34,33.12 | 72.34,33.12 v73.43,32.03 | 72.34,33.12 72.4,33.18 72.4,46.5
  Bottom 0.254: v73.5,21 v73.5,21.01 73.43,21.07 v73.43,32.03
HEATSINK  (via drill 0.7)
  other vias: 3.54,80.5 6.08,80.5 8.62,80.5 11.16,80.5 13.7,80.5 16.24,80.5 1,77.96 3.54,77.96 6.08,77.96 8.62,77.96 11.16,77.96 13.7,77.96 16.24,77.96 1,75.42 3.54,75.42 6.08,75.42 8.62,75.42 11.16,75.42 13.7,75.42 16.24,75.42 1,72.88 3.54,72.88 6.08,72.88 8.62,72.88 11.16,72.88 13.7,72.88 16.24,72.88 1,70.34 3.54,70.34 11.16,70.34 13.7,70.34 16.24,70.34 1,67.8 3.54,67.8 11.16,67.8 13.7,67.8 16.24,67.8 1,65.26 3.54,65.26 6.08,65.26 8.62,65.26 11.16,65.26 13.7,65.26 16.24,65.26 1,62.72 3.54,62.72 6.08,62.72 8.62,62.72 11.16,62.72 13.7,62.72 16.24,62.72 1,60.18 3.54,60.18 6.08,60.18 8.62,60.18 11.16,60.18 13.7,60.18 16.24,60.18 1,57.64 3.54,57.64 6.08,57.64 8.62,57.64 11.16,57.64 13.7,57.64 16.24,57.64 1,55.72 3.54,55.72 6.08,55.72 8.62,55.72 11.16,55.72 13.7,55.72 16.24,55.72 1.04,80.5
  pour Bottom: 0,82 17.7,82 17.7,54.8 0,54.8
  pour Top: 0,82 17.7,82 17.7,54.8 0,54.8
LED1_SIG  (via drill 0.6)
  Top 0.254: v47.57,36.98 47.04,36.45 36.47,36.45 35.99,35.97 U2.25
  Top 0.305: R3.1 v47.65,44.5
  Bottom 0.305: v47.65,44.5 47.65,37.06 v47.57,36.98
LED2_SIG  (via drill 0.6)
  Top 0.254: U2.12 15.67,45.85 16.1,46.28 v26.34,46.28 | v39.7,46 41.42,46 R2.1
  Bottom 0.254: v26.34,46.28 39.42,46.28 v39.7,46
MISO
  Bottom 0.305: ISP1.1 18.11,34.98 U2.18
MOSI  (via drill 0.6)
  Top 0.305: U2.17 13.46,32.77 9.83,32.77 9.73,32.66 9.73,24.16 v9.78,24.11
  Bottom 0.305: v9.78,24.11 9.78,21.57 ISP1.4
N$1
  Bottom 0.254: U2.9 23.29,46.51 Y1.2 24.82,51.39 C2.1
N$2
  Top 1.27: U$5.P$3 76.34,29.39 R6.1
N$3
  Bottom 0.254: U2.10 20.75,47.02 Y1.1 C1.1
N$4
  Bottom 0.305: C15.1 25.8,35.01 U2.21
N$5
  Top 0.254: R33.1 84.5,63.88 R22.1 91.3,63.66 U$2.4
N$6
  Top 0.305: LED2.A 43.1,46.01 R2.2
N$7
  Top 0.305: LED1.A 47.62,48.08 R3.2
N$10
  Top 0.254: U$5.P$1 76.01,24.31 76.35,24.65 76.35,26.42 R27.2
N$11
  Top 0.406: R21.2 20.21,83.18 U$9.CIRCUIT1
N$12
  Top 0.254: U2.24 37.72,30.71 R25.1
N$13  (via drill 0.6)
  Top 0.254: R28.1 71.24,20.76 73,19 74.12,19 R30.2 74.18,18.18 74.62,17.73 v78,17.73 | v82.68,17.73 88.09,17.73 89.53,16.28 89.53,12.93 89.89,12.58 IC2.2
  Bottom 0.254: v78,17.73 82.63,17.73 82.65,17.7 v82.68,17.73
N$14
  Bottom 0.254: R16.1 37.71,75.61 R19.2
N$15  (via drill 0.6)
  Top 0.305: IC3.2 34.85,25.7 v35.94,25.7
  Bottom 0.305: v35.94,25.7 37.76,25.7 C29.2
N$16
  Bottom 0.305: IC3.6 21.23,25.64
  Bottom 0.813: C31.2 21.23,25.64
N$17
  Bottom 0.254: R19.1 41.41,75.56 R20.2
N$18
  Top 0.254: R1.1 R12.2
  Top 0.305: R1.1 85.08,49.7 U$1.1 87.4,47.38 87.4,43.34 U$1.3
N$20
  Top 0.305: R30.1 76.47,19.65 R34.1 80.72,17.93 80.72,15.65 82.52,13.85 IC2.6
N$21
  Top 0.406: R5.2 22.7,85.7 25.5,88.5 34.5,88.5 35.5,87.5 35.5,85.44 U$3.CIRCUIT1
N$22
  Top 0.254: R31.2 R29.1 94.68,12.5 94.5,12.5 93.15,13.85 IC2.3
N$24  (via drill 0.6)
  Top 0.254: SJ1.2 65,84.5 v64.5,84
  Top 0.406: R32.1 24.95,83.05 v24.5,83.5 | v21,86.5 24,89.5 41.5,89.5 v43.5,87.5
  Bottom 0.254: v64.5,84 63.5,83 61.5,83 57.5,87 54.8,87 U$6.CIRCUIT1
  Bottom 0.406: v43.5,87.5 50.84,87.5 U$6.CIRCUIT1 | v21,86.5 21,84 21.5,83.5 v24.5,83.5
N$27  (via drill 1)
  other vias: 53.11,21.64
N$28  (via drill 1)
  other vias: 55.65,31.8
N$29  (via drill 1)
  other vias: 58.19,31.8
N$30  (via drill 1)
  other vias: 60.73,31.8
N$31  (via drill 1)
  other vias: 63.27,31.8
N$32  (via drill 1)
  other vias: 63.27,21.64
N$33  (via drill 1)
  other vias: 63.27,29.26
N$34  (via drill 1)
  other vias: 60.73,29.26
N$35  (via drill 1)
  other vias: 55.65,29.26
N$36  (via drill 1)
  other vias: 53.11,31.8 50.72,29.13 50.7,26.7 50.72,24.21
N$37  (via drill 1)
  other vias: 53.11,29.26
N$38  (via drill 1)
  other vias: 53.11,26.72
N$41  (via drill 1)
  other vias: 53.11,24.18
N$45  (via drill 1)
  other vias: 55.65,21.64
N$46  (via drill 1)
  other vias: 55.65,24.18
N$47  (via drill 1)
  other vias: 55.65,26.72
N$48  (via drill 1)
  other vias: 58.19,29.26
N$49  (via drill 1)
  other vias: 58.19,26.72
N$50  (via drill 1)
  other vias: 58.19,24.18
N$55  (via drill 1)
  other vias: 60.73,21.64
N$56  (via drill 1)
  other vias: 60.73,24.18
N$58  (via drill 1)
  other vias: 60.73,26.72
N$59  (via drill 1)
  other vias: 63.27,26.72
N$60  (via drill 1)
  other vias: 63.27,24.18
N$62
  Bottom 0.305: C21.1 23.21,38.33 L1.2 23.35,35.03 U2.20
N$63
  Bottom 0.305: C26.1 33.93,27.07 IC3.1
N$65
  Bottom 0.305: IC3.3 28.85,26.81 C26.2
N$66
  Bottom 0.305: IC3.4 26.31,25.74 C28.1
N$67
  Bottom 0.305: IC3.5 23.77,25.74 C28.2
P2  (via drill 1)
  other vias: 58.19,21.64
REMOTE_KILL  (via drill 0.6)
  Top 0.254: v42,57.5 v48,63.5 | v45.5,66.5 45.5,67.5 50,72 v50,72.5 | U$6.CIRCUIT2 48.93,86.93 51.5,89.5 57,89.5 v59,91.5 | v65,89.5 65,88 | 65,88 SJ1.1 | U$8.4 78.36,84.14 v78,84.5 | 65,88 66,89 67.6,89 v68,89.4 | v45,81 45,77.9 v48,74.9
  Bottom 0.254: v48,63.5 48,64 v45.5,66.5 | v45,81 45,81.34 U$6.CIRCUIT2 | v59,91.5 64,91.5 65,90.5 v65,89.5 | v78,84.5 73,89.5 68.1,89.5 v68,89.4 | v50,72.5 50,72.9 v48,74.9 | U2.11 18.21,48.69 15.9,51 15.9,51.69 17.3,53.09 37.59,53.09 v42,57.5
  Bottom 0.305: R37.1 18.21,41.16 U2.11
RXD
  Bottom 0.254: U2.2 41.07,37.21 39.85,35.99 39.85,33.83 35.84,29.82 35.84,27.43 33.76,25.35 33.76,23.88 33.38,23.5 25.73,23.5 IC3.12
  Bottom 0.305: JP6.P$3 2.31,37.19 2.31,14.48 2.74,14.05 8.41,14.05 13.41,19.05 22.76,19.05 23.77,20.07 IC3.12
RXD_LOG
  Top 0.254: U2.15 16.46,40.84 46.28,40.84 49.49,44.05 JP2.3
RXD_OUT
  Bottom 0.305: IC3.13 26.31,15.8 26.77,15.34 26.77,11.28 26.67,11.18 26.24,11.18 25.3,10.24 25.3,8.26 26.95,6.6 30.22,6.6 COMMS_ETH.P$3
SCK
  Bottom 0.305: ISP1.3 5.61,19.68 5.61,21.57 17.68,33.63 19.41,33.63 U2.19
SCL
  Top 0.254: CN1.4 57.05,35 56.54,34.49 51.18,34.49 49.51,32.82 45.77,32.82 U2.28
SDA
  Top 0.254: U2.27 41.07,32.66 41.6,32.13 49.91,32.13 51.54,33.76 58.01,33.76 58.17,33.91 58.17,78.05 58.67,78.56 58.67,79.78 58.55,79.91 55.7,79.91 CN1.3
TARE  (via drill 0.6)
  Top 0.305: S2.1 70.32,96.01 48.34,96.01 45.03,92.71 45.03,84.73 44.96,84.73 v44.93,84.76 | v40.34,77.42 40.34,56.57 v34.11,50.34 | v28.14,49.94 15.47,49.94 13.13,47.6 U2.13
  Top 0.406: S2.1 S2.2
  Bottom 0.305: U2.13 13.19,42.54 R8.1 | v44.93,84.76 40.39,80.21 40.39,77.47 v40.34,77.42 | v34.11,50.34 28.55,50.34 v28.14,49.94
TXD  (via drill 0.6)
  Top 0.254: IC3.11 27.69,27.99 27.69,30.61 28.75,31.67 v35,31.67
  Bottom 0.254: v35,31.67 35.08,31.67 37.29,33.88 37.29,36.42 38.56,37.69 38.56,42.57 U2.3
  Bottom 0.305: JP6.P$2 2.87,35.2 2.87,14.91 3.12,14.66 8.08,14.66 13.06,19.63 20.75,19.63 21.23,20.12 IC3.11
TXD_LOG  (via drill 0.6)
  Top 0.254: U2.16 18.39,40.23 46.69,40.23 47.6,41.15 48.28,41.15 48.31,41.15 49,41.15 v48.79,41.35
  Bottom 0.254: v48.79,41.35 49.66,42.22 49.66,45.58 JP2.2
TXD_OUT
  Bottom 0.305: IC3.14 28.85,10.08 COMMS_ETH.P$6
V_ADJ
  Top 0.406: IC1.1 24.8,71.2 26,70 D2.A
  Bottom 0.203: R17.1 34.06,81.46 R18.2 R16.2
  Bottom 0.254: R15.1 34.06,75.66 R16.2 34.11,72.34 R14.1 34.1,72.25 32.5,72.25 | R13.1 32.5,72.25 | 32.5,72.25 32.5,71.5 32.2,71.2 28.3,71.2 27.5,72 22.8,72 22.3,71.5 IC1.1 21,72.2 C9.1
WB_ARM1
  Top 0.254: U$4.3 U$4.4 94.96,22.18 R29.2
WB_ARM2
  Top 0.254: U$5.P$2 69.85,26.85 69,26 69,20.89 R28.2

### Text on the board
tPlace: Reset | Tare | Config | Remote Kill Override | ESTOP1 | ESTOP2 | Remote Kill | 7-segment Display | WARNING: Solder only / one H2 sensor and its / components on each / PCB. / Refer documentation. | IDT SGAS 701 | Note: This board has multiple / configuration options and / specific rules for / operation. / Please read the documentation / carefully before soldering / and operating this board. | MQ-8 | Sparkfun Openlog | Figaro TGS6812 | Protoboard | Wheatstone Bridge Arms / Multimeter Probe Points | Arm2 | Arm1 | FCC_ETH
bPlace: WARNING: Solder only one / branch of resistors / on each PCB. / Refer / documentation. | Figaro | Figaro | C:/EAGLE-7.6.0/ulp/bw_bmp_chem_cat.bmp | IDT | MQ-8 | Ordered: YYYY/MM/DD

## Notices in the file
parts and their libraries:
SparkFun-DigitalIC: Licensing: Creative Commons ShareAlike 4.0 International - https://creativecommons.org/licenses/by-sa/4.0
SparkFun: Licensing: CC v3.0 Share-Alike You are welcome to use this library for commercial purposes.
